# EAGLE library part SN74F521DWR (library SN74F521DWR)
8-Bit Identity/Magnitude Comparators (P=Q) with Enable Source: Datasheet
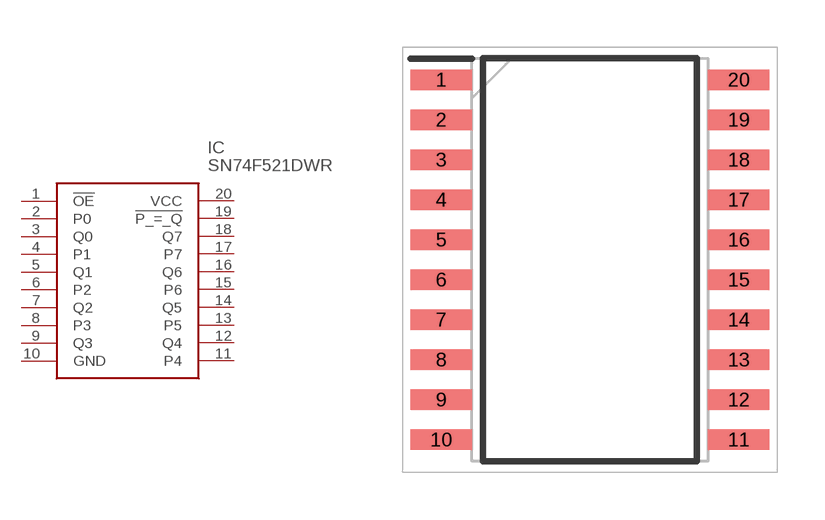
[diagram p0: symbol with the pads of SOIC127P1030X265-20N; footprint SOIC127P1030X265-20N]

Designator prefix IC

## SN74F521DWR (Description: 8-Bit Identity/Magnitude Comparators (P=Q) with Enable; Height: 2.65mm; Manufacturer_Name: Texas Instruments; Manufacturer_Part_Number: SN74F521DWR; Mouser_Part_Number: 595-SN74F521DWR; Mouser_Price-Stock: https://www.mouser.co.uk/ProductDetail/Texas-Instruments/SN74F521DWR?qs=mE33ZKBHyE6Hxf0oNfiDUg%3D%3D)  [SOIC127P1030X265-20N]
1  !OE
2  P0
3  Q0
4  P1
5  Q1
6  P2
7  Q2
8  P3
9  Q3
10  GND
11  P4
12  Q4
13  P5
14  Q5
15  P6
16  Q6
17  P7
18  Q7
19  !P_=_Q
20  VCC

## Footprint SOIC127P1030X265-20N (pad centres in mm)
DW0020A
smd 1.95 x 0.65: 1 -4.725,5.715; 2 -4.725,4.445; 3 -4.725,3.175; 4 -4.725,1.905; 5 -4.725,0.635; 6 -4.725,-0.635; 7 -4.725,-1.905; 8 -4.725,-3.175; 9 -4.725,-4.445; 10 -4.725,-5.715; 11 4.725,-5.715; 12 4.725,-4.445; 13 4.725,-3.175; 14 4.725,-1.905; 15 4.725,-0.635; 16 4.725,0.635; 17 4.725,1.905; 18 4.725,3.175; 19 4.725,4.445; 20 4.725,5.715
